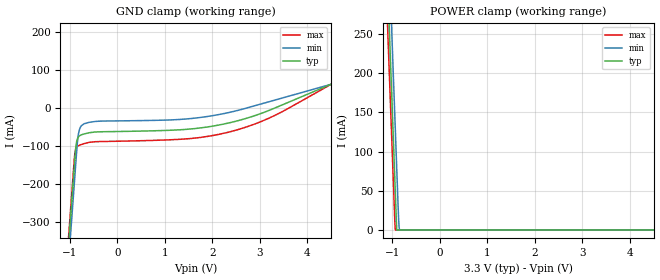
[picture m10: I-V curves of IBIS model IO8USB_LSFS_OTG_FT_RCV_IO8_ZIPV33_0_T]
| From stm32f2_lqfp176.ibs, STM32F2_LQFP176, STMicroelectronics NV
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| *** New cell (Generated with 5.14beta1 (Sep 20 2010 13:23:23))
[Model]   IO8USB_LSFS_OTG_FT_RCV_IO8_ZIPV33_0_T
Model_type Input
Polarity   Non-Inverting
Enable   Active-Low
| CAP_THRESHOLD on pad DPV33 is "CMOS" :
| Rising=10.0% of vddio   Falling=90.0% of vddio
| C_comp min and max val. don't necessarily correlate with the min and max pvt
| but are the smallest and greatest pad capacitance found.
| var   typ   min   max
C_comp   1.93475pF  1.87905pF  1.99935pF
Vinl = 800.0mV | Dummy value overriden by next lines
Vinh = 2.00V | Dummy value overriden by next lines
[Model Spec]
| TIME_THRESHOLD on pin ZIPV33 is "CORE" :
| Rising=40.0% of vddio   Falling=60.0% of vddio
Vinl 1.25450V 1.03850V 1.36250V
Vinh 1.66150V 1.36950V 1.82450V
| variable   typ   min   max
[Temperature Range] 25.0 125.0 -40.0
| variable   typ   min   max
[Voltage Range] 3.3V 2.7V 3.6V
| variable   typ   min   max
[POWER Clamp Reference] 3.3V 2.7V 3.6V
| variable   typ   min   max
[GND Clamp Reference] 0V 0V 0V
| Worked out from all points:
|   POWER clamp passes 1 mA (typ) near -0.91 V on its own axis
[POWER Clamp]
-3.3V     3.936A     4.058A     3.841A
-1.13V    361.8mA    445mA      304.1mA
-1.09V    295.9mA    378.4mA    238.9mA
-1.05V    230mA      311.8mA    173.7mA
-1.01V    164.1mA    245.2mA    108.5mA
-950mV    65.28mA    145.3mA    10.76mA
-940mV    48.81mA    128.7mA    0A
-910mV    0A         78.72mA    0A
-870mV    0A         14.2mA     0A
-860mV    0A         3.389mA    0A
-850mV    0A         0A         0A
6.6V      0A         0A         0A
[GND Clamp]
-3.3V     -4.218A    -4.264A    -4.198A
-1.06V    -410mA     -456mA     -390.4mA
-940mV    -206mA     -252mA     -186.4mA
-890mV    -121mA     -167mA     -113.8mA
-860mV    -88.28mA   -116mA     -102.8mA
-820mV    -75.08mA   -66.92mA   -98.42mA
-780mV    -70.94mA   -49.85mA   -96.22mA
-700mV    -67.36mA   -40.52mA   -92.83mA
1.65V     -53.05mA   -25.58mA   -78.06mA
2.72V     -26.13mA   701.5uA    -48.88mA
3.54V     12.65mA    29.46mA    -4.159mA
6.6V      173.9mA    136.8mA    210.6mA
